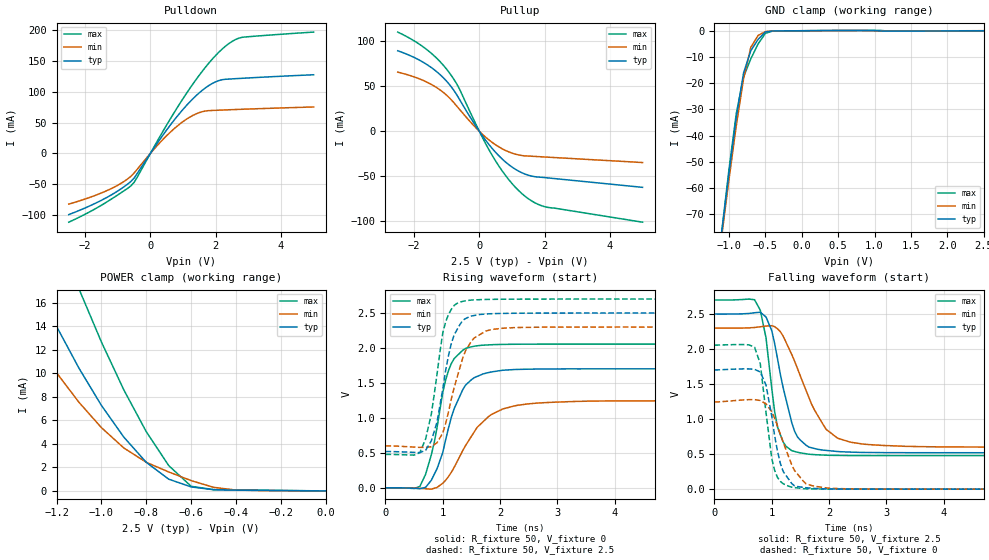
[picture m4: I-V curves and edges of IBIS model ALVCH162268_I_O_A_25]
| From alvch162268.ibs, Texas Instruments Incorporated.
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|************* ALVCH162268 OUTPUT (2.5 V) MODEL**************
[Model]   ALVCH162268_I_O_A_25
Model_type  I/O
Polarity   Non-Inverting
Enable   Active-Low
Vinl = 0.7V
Vinh = 1.7V
Vmeas = 1.25V
Cref = 30pF
Rref = 500
Vref = 0
| variable   typ   min   max
C_comp   8.15pF   NA   NA
[Temperature Range]   50   100   0
[Voltage range]   2.5   2.3   2.7
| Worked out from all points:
|   slope of the pulldown table from 0 to 0.375 V, typ, clamps not added: 12.9 ohm
|   slope of the pullup table from 0 to 0.375 V, typ, clamps not added: 20.6 ohm
|   GND clamp passes 1 mA (typ) near -0.52 V on its own axis
|   POWER clamp passes 1 mA (typ) near -0.70 V on its own axis
|   rising waveform, R_fixture 50, V_fixture 0: 20-80 % time 396ps typ, 601ps min, 310ps max; typ from 0 V to 1.7 V
|   falling waveform, R_fixture 50, V_fixture 2.5: 20-80 % time 319ps typ, 557ps min, 217ps max; typ from 2.5 V to 0.52 V
|   rising waveform, R_fixture 50, V_fixture 2.5: 20-80 % time 275ps typ, 341ps min, 249ps max; typ from 0.52 V to 2.5 V
|   falling waveform, R_fixture 50, V_fixture 0: 20-80 % time 234ps typ, 358ps min, 187ps max; typ from 1.7 V to 0 V
|Process range|   weak   strong
[Pullup]
|   50C:2.5V:   100C:2.3V:weak   0C:2.7V:strong
|   Voltage   I(typ)   I(min)   I(max)
-2.5V     89.46mA    65.74mA    110.2mA
-1.7V     76.26mA    56.19mA    93.25mA
-1.3V     66.04mA    48.37mA    80.96mA
-1V       55.55mA    40.05mA    68.91mA
-600mV    35mA       24.11mA    46.42mA
0V        0A         0A         0A
400mV     -19.31mA   -12.5mA    -27.07mA
900mV     -36.99mA   -22.83mA   -53.62mA
1.4V      -47.51mA   -27.29mA   -72.11mA
1.7V      -50.39mA   -27.89mA   -79.34mA
2.1V      -51.75mA   -28.72mA   -84.5mA
5V        -62.22mA   -34.67mA   -100.9mA
[Pulldown]
|   50C:2.5V:   100C:2.3V:weak   0C:2.7V:strong
|   Voltage   I(typ)   I(min)   I(max)
-2.5V     -99.33mA   -82.25mA   -111.6mA
-1.2V     -67.47mA   -57.11mA   -74.25mA
-800mV    -53.83mA   -45.25mA   -60.34mA
-500mV    -40.21mA   -31.89mA   -47.11mA
400mV     30.84mA    23.5mA     37.25mA
1.1V      77.46mA    55.35mA    96.99mA
1.5V      98.47mA    66.26mA    127.1mA
1.8V      110.5mA    69.5mA     147.1mA
2.3V      120.3mA    70.62mA    174mA
2.6V      121.3mA    71.24mA    184.6mA
2.8V      121.9mA    71.64mA    188.3mA
5V        127.7mA    75.38mA    196.9mA
[GND Clamp]
|   50C:2.5V:   100C:2.3V:weak   0C:2.7V:strong
|   Voltage   I(typ)   I(min)   I(max)
-2.5V     -430mA     -414.8mA   -445.7mA
-1.1V     -77.02mA   -78.47mA   -76.66mA
-1V       -54.25mA   -56.74mA   -52.91mA
-900mV    -33.13mA   -36.27mA   -31.6mA
-800mV    -16.14mA   -18.34mA   -17.63mA
-700mV    -7.586mA   -6.301mA   -10.71mA
-600mV    -3.292mA   -1.788mA   -5mA
-500mV    -442.6uA   -314.5uA   -1.009mA
-400mV    -86.82uA   -82.8uA    -114.9uA
800mV     108.5uA    63.96uA    161.5uA
1.2V      -120uA     -68.18uA   -179uA
2.5V      123.5pA    21.94uA    -39.79uA
[POWER Clamp]
|   50C:2.5V:   100C:2.3V:weak   0C:2.7V:strong
|   Voltage   I(typ)   I(min)   I(max)
-2.5V     80.46mA    60.73mA    105.4mA
-1.5V     26.54mA    19.28mA    38.52mA
-1.4V     22.09mA    15.96mA    32.77mA
-1.3V     17.89mA    12.87mA    27.27mA
-1.2V     14mA       10.05mA    22.06mA
-1.1V     10.44mA    7.536mA    17.18mA
-900mV    4.57mA     3.651mA    8.587mA
-800mV    2.429mA    2.433mA    5.033mA
-700mV    998.3uA    1.613mA    2.154mA
-600mV    341.9uA    876.7uA    391.3uA
-400mV    66.77uA    70.77uA    86.75uA
0V        121.4pA    549.5pA    66.34pA
[ramp]
| variable   typ   min   max
dV/dt_r   1.0286E+00/3.9920E-10  7.5794E-01/6.0531E-10  1.2389E+00/3.0842E-10
dV/dt_f   1.2030E+00/3.1822E-10  1.0396E+00/5.6668E-10  1.3405E+00/2.1855E-10
[Rising Waveform]
R_fixture = 50
V_fixture = 0
V_fixture_min = 0
V_fixture_max = 0
C_fixture = 0
L_fixture = 0
|   50C:2.5V:   100C:2.3V:weak   0C:2.7V:strong
|   Time   V(typ)   V(min)   V(max)
0s        0V         0V         0V
600ps     -11.75mV   -6.103mV   21.02mV
800ps     109.5mV    -17.98mV   473.4mV
900ps     274.1mV    7.043mV    863.5mV
1.1ns     857.7mV    162.8mV    1.677V
1.35ns    1.407V     536.6mV    1.97V
1.55ns    1.577V     802.1mV    2.026V
2.05ns    1.682V     1.129V     2.052V
2.9ns     1.701V     1.224V     2.056V
13.5ns    1.702V     1.245V     2.056V
[Falling Waveform]
R_fixture = 50
V_fixture = 2.5
V_fixture_min = 2.3
V_fixture_max = 2.7
C_fixture = 0
L_fixture = 0
|   50C:2.5V:   100C:2.3V:weak   0C:2.7V:strong
|   Time   V(typ)   V(min)   V(max)
0s        2.5V       2.3V       2.7V
700ps     2.517V     2.307V     2.703V
800ps     2.525V     2.317V     2.554V
900ps     2.458V     2.327V     2.16V
1.1ns     1.865V     2.289V     887.9mV
1.35ns    946.9mV    1.92V      549.4mV
1.5ns     699.3mV    1.614V     517.5mV
1.95ns    552.8mV    853.1mV    484.7mV
2.6ns     523.9mV    642.5mV    479.4mV
13.5ns    519.6mV    600mV      478.5mV
[Rising Waveform]
R_fixture = 50
V_fixture = 2.5
V_fixture_min = 2.3
V_fixture_max = 2.7
C_fixture = 0
L_fixture = 0
|   50C:2.5V:   100C:2.3V:weak   0C:2.7V:strong
|   Time   V(typ)   V(min)   V(max)
0s        519.6mV    600mV      478.5mV
500ps     508mV      583.6mV    469mV
700ps     536.3mV    579.3mV    698.4mV
900ps     943mV      647.1mV    1.628V
1.05ns    1.681V     920mV      2.373V
1.2ns     2.191V     1.439V     2.61V
1.4ns     2.422V     1.966V     2.676V
1.75ns    2.486V     2.242V     2.695V
2.3ns     2.497V     2.293V     2.699V
13.5ns    2.5V       2.3V       2.7V
[Falling Waveform]
R_fixture = 50
V_fixture = 0
V_fixture_min = 0
V_fixture_max = 0
C_fixture = 0
L_fixture = 0
|   50C:2.5V:   100C:2.3V:weak   0C:2.7V:strong
|   Time   V(typ)   V(min)   V(max)
0s        1.702V     1.245V     2.056V
700ps     1.709V     1.278V     2.026V
800ps     1.673V     1.265V     1.79V
900ps     1.485V     1.217V     1.093V
1.05ns    764.1mV    1.013V     270.5mV
1.2ns     251.8mV    668.6mV    77.35mV
1.35ns    78.85mV    343.7mV    27.64mV
1.6ns     19.95mV    76.38mV    5.091mV
2.15ns    1.942mV    8.509mV    859.8uV
13.5ns    -1.407uV   2.101uV    821.5nV
